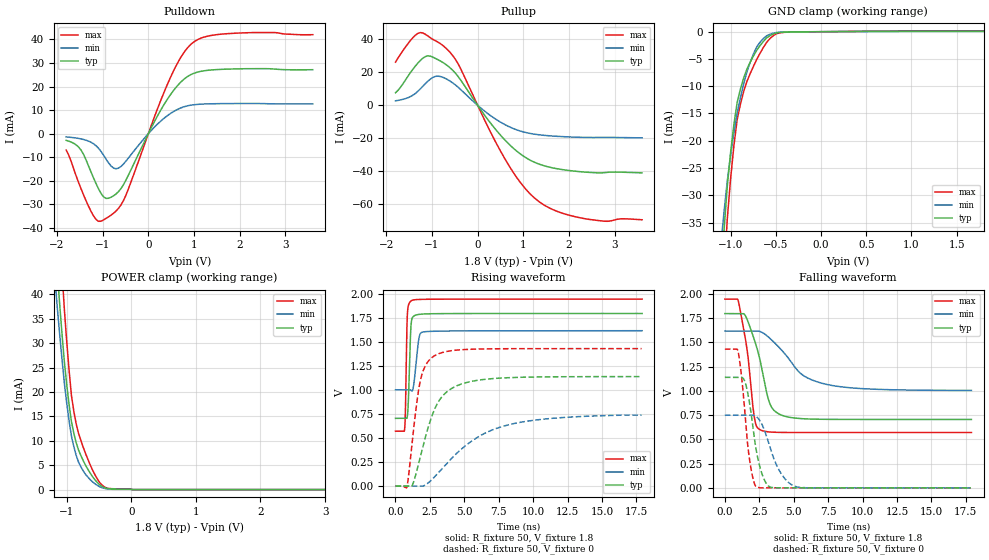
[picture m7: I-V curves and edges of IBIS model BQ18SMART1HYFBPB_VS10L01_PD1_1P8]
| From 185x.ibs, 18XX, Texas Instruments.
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|   Model Cell BQ18SMART1HYFBPB_VS10L01_PD1_1P8
|BQ18SMART1HYFBPB_VS10L01_PD1_1P8
[Model]   BQ18SMART1HYFBPB_VS10L01_PD1_1P8
Model_type   I/O
Polarity   Non-Inverting
Enable   Active-Low
Vinl =  0.63
Vinh =  1.17
Cref =  15pF
Rref =  100.0000M
Vref =  0V
Vmeas =  0.9
C_comp   0.9029199p   0.7983694p   1.014934p
[Model Spec]
Vinl   0.63   0.567   0.6825
Vinh   1.17   1.053   1.2675
[Temperature Range]   25   125   -40
[Voltage Range]   1.8   1.62   1.95
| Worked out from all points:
|   slope of the pulldown table from 0 to 0.27 V, typ, clamps not added: 27.2 ohm
|   slope of the pullup table from 0 to 0.27 V, typ, clamps not added: 26 ohm
|   GND clamp passes 1 mA (typ) near -0.59 V on its own axis
|   POWER clamp passes 1 mA (typ) near -0.49 V on its own axis
|   rising waveform, R_fixture 50, V_fixture 1.8: 20-80 % time 147ps typ, 270ps min, 102ps max; typ from 0.706 V to 1.8 V
|   rising waveform, R_fixture 50, V_fixture 0: 20-80 % time 1.61ns typ, 3.98ns min, 799ps max; typ from 0 V to 1.14 V
|   falling waveform, R_fixture 50, V_fixture 1.8: 20-80 % time 1.12ns typ, 2.48ns min, 708ps max; typ from 1.8 V to 0.706 V
|   falling waveform, R_fixture 50, V_fixture 0: 20-80 % time 771ps typ, 1.22ns min, 583ps max; typ from 1.14 V to 0 V
| Nom Voltages:
|   BIASFET=1.8, VBBNW=1.1, VDD=1.1, VDDS=1.8, VSS=0, VSSS=0
| Min Voltages:
|   BIASFET=1.62, VBBNW=0.99, VDD=0.99, VDDS=1.62, VSS=0, VSSS=0
| Max Voltages:
|   BIASFET=1.95, VBBNW=1.21, VDD=1.21, VDDS=1.95, VSS=0, VSSS=0
[POWER_clamp]
|   voltage   I(typ)   I(min)   I(max)
-1.8V     196.9mA    157.5mA    250.4mA
-1.182V   51.67mA    43mA       68.61mA
-1.145V   44.45mA    37.16mA    60.1mA
-1.109V   37.9mA     31.74mA    52.07mA
-1.073V   31.79mA    26.6mA     44.33mA
-1.036V   26.12mA    21.74mA    36.87mA
-963.6mV  17.39mA    14.07mA    24.42mA
-927.3mV  13.91mA    10.96mA    19.29mA
-854.5mV  9.657mA    7.054mA    13.5mA
-709.1mV  4.995mA    3.131mA    7.393mA
-490.9mV  991uA      585.4uA    1.466mA
3.6V      0A         0A         0A
[Pulldown]
|   voltage   I(typ)   I(min)   I(max)
-1.8V     -2.835mA   -1.376mA   -6.938mA
-1.473V   -6.994mA   -2.229mA   -23.44mA
-1.2V     -18.79mA   -4.282mA   -34.89mA
-1.036V   -25.34mA   -7.531mA   -37.14mA
-872.7mV  -27.39mA   -12.36mA   -35.28mA
-654.5mV  -24.59mA   -14.63mA   -31.68mA
-490.9mV  -19.69mA   -11.65mA   -26.08mA
381.8mV   13.54mA    7.116mA    19.32mA
654.5mV   20.72mA    10.44mA    30.47mA
927.3mV   25mA       12.07mA    37.79mA
1.636V    27.3mA     12.74mA    42.26mA
3.6V      27.12mA    12.64mA    41.97mA
[Pullup]
|   voltage   I(typ)   I(min)   I(max)
-1.8V     7.614mA    2.74mA     26.22mA
-1.527V   17.69mA    4.626mA    37.43mA
-1.309V   25.69mA    8.541mA    43.72mA
-1.036V   29.87mA    15.94mA    41.05mA
-818.2mV  26.95mA    17.52mA    37.49mA
-490.9mV  19.61mA    12.45mA    28.08mA
545.5mV   -19.54mA   -10.94mA   -30.03mA
927.3mV   -29.38mA   -15.56mA   -46.58mA
1.255V    -34.7mA    -17.56mA   -56.51mA
1.691V    -38.25mA   -18.74mA   -63.85mA
2.291V    -40.42mA   -19.45mA   -68.55mA
3.6V      -41.01mA   -19.75mA   -69.5mA
[GND_clamp]
|   voltage   I(typ)   I(min)   I(max)
-1.8V     -274mA     -200.4mA   -365.5mA
-1.109V   -45.41mA   -39.33mA   -55.91mA
-1.073V   -36.49mA   -33.11mA   -44.46mA
-1.036V   -28.34mA   -27.37mA   -34.29mA
-1V       -22.19mA   -22.71mA   -27mA
-927.3mV  -12.97mA   -14.93mA   -16.12mA
-854.5mV  -8.452mA   -9.555mA   -10.93mA
-781.8mV  -5.549mA   -5.539mA   -7.634mA
-709.1mV  -3.363mA   -2.741mA   -5.028mA
-600mV    -1.121mA   -737.1uA   -1.924mA
-381.8mV  -62.21uA   -38.42uA   -93.33uA
1.8V      98.66uA    51.35uA    168.2uA
[Ramp]
| variable   typ   min   max
dV/dt_f 0.65718224/1.1239422n 0.37039334/2.5000018n 0.82808182/0.71153767n
dV/dt_r 0.69623206/1.6153088n 0.45769507/4.1471966n 0.87036834/0.80278996n
R_load = 50
[Rising Waveform]
R_fixture = 50
V_fixture = 1.8
V_fixture_min = 1.62
V_fixture_max = 1.95
|   time   V(typ)   V(min)   V(max)
0s        705.7mV    1.003V     572mV
659.2ps   705.7mV    1.003V     588.4mV
718.1ps   705.7mV    1.003V     763.8mV
814.9ps   705.7mV    1.003V     1.56V
863.4ps   730.7mV    1.003V     1.792V
1.099ns   1.602V     1.002V     1.926V
1.177ns   1.733V     990.7mV    1.934V
1.709ns   1.789V     1.545V     1.945V
1.954ns   1.792V     1.604V     1.946V
17.91ns   1.798V     1.619V     1.948V
[Rising Waveform]
R_fixture = 50
V_fixture = 0
V_fixture_min = 0
V_fixture_max = 0
|   time   V(typ)   V(min)   V(max)
0s        0V         0V         0V
827.3ps   0V         0V         -10.26mV
1.196ns   0V         0V         435.4mV
1.543ns   157.1mV    0V         865.9mV
1.795ns   301.4mV    0V         1.091V
2.178ns   514mV      12.71mV    1.255V
2.863ns   807.9mV    100.1mV    1.36V
4.41ns    1.042V     336.3mV    1.416V
7.724ns   1.126V     619.5mV    1.431V
17.87ns   1.141V     739.3mV    1.432V
[Falling Waveform]
R_fixture = 50
V_fixture = 1.8
V_fixture_min = 1.62
V_fixture_max = 1.95
|   time   V(typ)   V(min)   V(max)
0s        1.798V     1.618V     1.947V
981ps     1.798V     1.618V     1.926V
1.619ns   1.738V     1.618V     1.423V
2.153ns   1.524V     1.618V     720.4mV
2.574ns   1.308V     1.612V     598.4mV
3.297ns   859.8mV    1.54V      575.9mV
4.368ns   738.4mV    1.382V     571.5mV
5.631ns   713.5mV    1.166V     571mV
7.57ns    706.7mV    1.062V     571mV
17.91ns   705.8mV    1.005V     571mV
[Falling Waveform]
R_fixture = 50
V_fixture = 0
V_fixture_min = 0
V_fixture_max = 0
|   time   V(typ)   V(min)   V(max)
0s        1.14V      749.8mV    1.431V
965.2ps   1.14V      749.8mV    1.405V
1.257ns   1.138V     749.8mV    1.093V
1.563ns   1.044V     749.8mV    589.8mV
1.914ns   763.5mV    749.8mV    185.8mV
2.301ns   372.5mV    733.2mV    7.089mV
3.146ns   21.96mV    480mV      0V
4.021ns   0V         163.2mV    0V
5.082ns   0V         16.3mV     0V
17.87ns   0V         0V         0V
